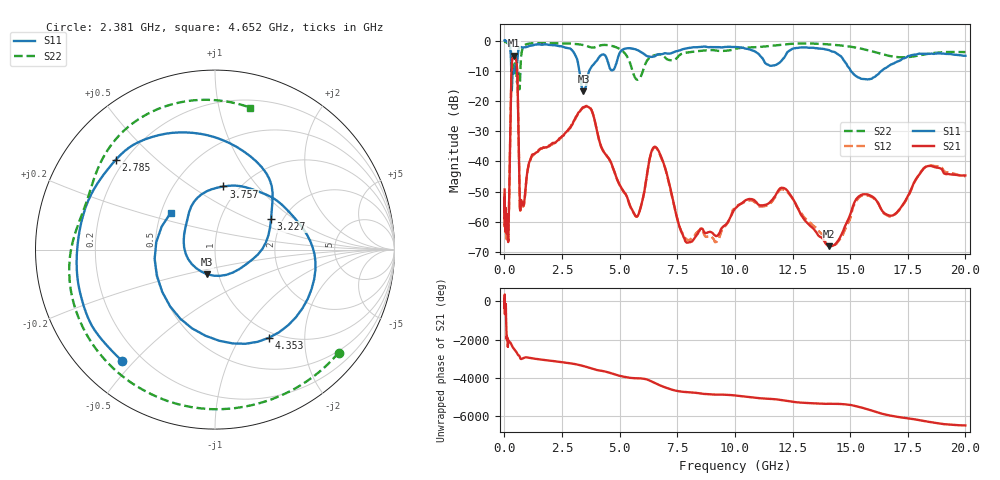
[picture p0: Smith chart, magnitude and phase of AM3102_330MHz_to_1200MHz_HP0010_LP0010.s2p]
! Date/Time: Tue, Sep 11, 2018 5:10 PM
! Network Analyzer: Agilent Technologies E8362B Rev: A.07.50.63
! Sweep from 0.010 to 20.000 GHz, 1601 Points, Sweep Type: LOG
! Power Supply: 4.950 V, 0.001 A
# Hz S DB R 50
!freq MagS11 AngS11 MagS21 AngS21 MagS12 AngS12 MagS22 AngS22
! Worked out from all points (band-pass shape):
!   1601 points, 10 MHz to 20 GHz, reference 50 ohm
!   highest |S21| = -4.99 dB at 406.7 MHz (marker M1); lowest = -68.1 dB at 14.07 GHz (marker M2)
!   |S21| within 3 dB of the highest: 320.9 MHz to 536.7 MHz (215.8 MHz wide, 50.3 % of centre)
!   lowest |S11| = -16.8 dB at 3.432 GHz (marker M3), VSWR 1.34, Z = 44.2 - j12.4 ohm
!   |S11| at or under -10 dB: 297.8 MHz to 361.6 MHz (63.73 MHz wide, 19.3 % of centre); 3.252 GHz to 3.684 GHz (431.5 MHz wide, 12.4 % of centre); 15.03 GHz to 16.37 GHz (1.347 GHz wide, 8.58 % of centre)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
!   |S22| runs from -16.2 to -0.2 dB; largest |S21 - S12| = 0.0084
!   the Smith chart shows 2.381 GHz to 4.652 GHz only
!   S11 on the Smith chart (normalised r, x): 2.381 GHz: 0.13, -0.46; 2.785 GHz: 0.17, +0.38; 3.227 GHz: 1.74, +0.68; 3.757 GHz: 0.85, +0.68; 4.353 GHz: 0.91, -1.34; 4.652 GHz: 0.56, +0.26
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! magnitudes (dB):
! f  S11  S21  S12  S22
! 10 MHz  0.0  -49.3  -50.6  -0.2
! 35.55 MHz  0.0  -62.3  -59.9  -0.4
! 126.4 MHz  -0.4  -62.2  -62.1  -0.8
! 190.2 MHz  -1.1  -58.7  -60.0  -1.2
! 406.7 MHz  -11.0  -5.0  -5.0  -8.6
! 447.2 MHz  -9.2  -5.3  -5.4  -7.6
! 559.1 MHz  -6.9  -11.2  -11.3  -13.5
! 685.8 MHz  -2.3  -56.3  -56.7  -12.2
! 1.59 GHz  -1.4  -35.8  -35.8  -0.9
! 2.381 GHz  -1.9  -32.4  -32.8  -0.9
! 2.785 GHz  -2.6  -29.4  -29.4  -1.0
! 3.227 GHz  -9.0  -23.8  -24.0  -1.3
! 3.432 GHz  -16.8  -22.0  -22.2  -1.5
! 3.757 GHz  -9.0  -22.7  -22.7  -2.3
! 4.353 GHz  -4.8  -37.3  -37.2  -1.5
! 4.652 GHz  -9.9  -40.9  -41.0  -1.8
! 5.652 GHz  -2.9  -57.7  -57.7  -12.1
! 6.58 GHz  -5.0  -35.4  -35.6  -4.8
! 7.92 GHz  -2.6  -66.9  -66.0  -4.0
! 12.09 GHz  -6.1  -48.8  -49.3  -1.3
! 14.07 GHz  -3.2  -68.1  -67.6  -1.3
! 20 GHz  -5.0  -44.7  -45.0  -3.8
